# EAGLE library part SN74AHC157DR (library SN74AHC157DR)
Quadruple 2-Line To 1-Line Data Selectors / Multiplexers Source: Datasheet
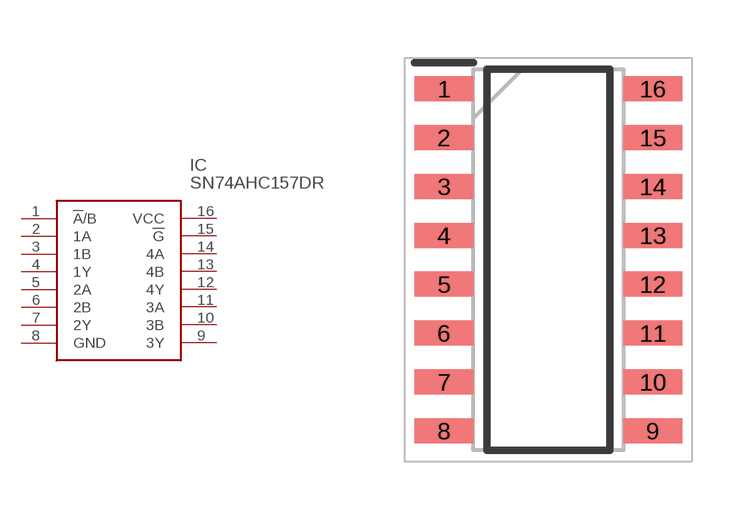
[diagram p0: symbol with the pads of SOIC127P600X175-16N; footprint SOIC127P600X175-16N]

Designator prefix IC

## SN74AHC157DR (Description: Quadruple 2-Line To 1-Line Data Selectors / Multiplexers; Height: 1.75mm; Manufacturer_Name: Texas Instruments; Manufacturer_Part_Number: SN74AHC157DR; Mouser_Part_Number: 595-SN74AHC157DR; Mouser_Price-Stock: https://www.mouser.co.uk/ProductDetail/Texas-Instruments/SN74AHC157DR?qs=nMmhAzRCgdCMVxhGfqxf9A%3D%3D)  [SOIC127P600X175-16N]
1  !A!/B  in
2  1A  in
3  1B  in
4  1Y  out
5  2A  in
6  2B  in
7  2Y  out
8  GND  pwr
9  3Y  out
10  3B  in
11  3A  in
12  4Y  out
13  4B  in
14  4A  in
15  !G  in
16  VCC  pwr

## Footprint SOIC127P600X175-16N (pad centres in mm)
D (R-PDSO-G16)
smd 1.525 x 0.65: 1 -2.712,4.445; 2 -2.712,3.175; 3 -2.712,1.905; 4 -2.712,0.635; 5 -2.712,-0.635; 6 -2.712,-1.905; 7 -2.712,-3.175; 8 -2.712,-4.445; 9 2.712,-4.445; 10 2.712,-3.175; 11 2.712,-1.905; 12 2.712,-0.635; 13 2.712,0.635; 14 2.712,1.905; 15 2.712,3.175; 16 2.712,4.445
